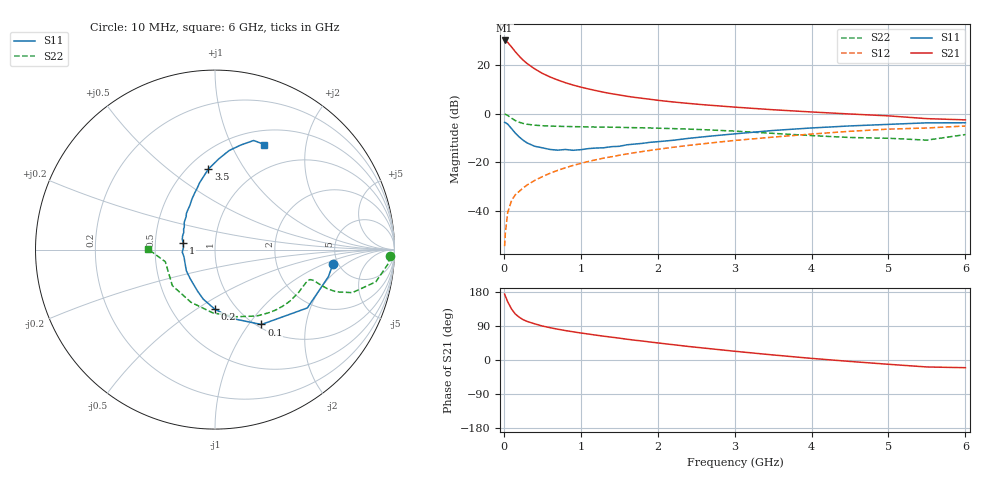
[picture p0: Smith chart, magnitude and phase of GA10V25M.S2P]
! Infineon Technologies  Discrete & RF Semiconductors
! BF775
! Si NPN RF Bipolar Junction Transistor in SOT23
! VCE = 10 V  IC = 25 mA
! Common Emitter S-Parameters:  May  1996
# GHz  S  MA  R  50
!  f  S11  S21  S12  S22
! GHz  MAG  ANG  MAG  ANG  MAG  ANG  MAG  ANG
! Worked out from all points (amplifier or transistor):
!   36 points, 10 MHz to 6 GHz, reference 50 ohm
!   highest |S21| = 30.0 dB at 10 MHz (marker M1)
!   |S21| within 3 dB of that: start of sweep to 108.8 MHz
!   unconditionally stable (mu >= 1): 401.8 MHz to 2.59 GHz
!   at 250 MHz: K = 0.86, MSG = 26.2 dB, |S12| = -30.5 dB
!   at 1.4 GHz: K = 1.10, MAG = 11.0 dB, |S12| = -17.7 dB
!   at 6 GHz: K = 0.90, MSG = 1.3 dB, |S12| = -5.1 dB
!   S11 on the Smith chart (normalised r, x): 10 MHz: 4.54, -1.29; 100 MHz: 1.05, -1.15; 200 MHz: 0.80, -0.59; 1 GHz: 0.70, +0.05; 3.5 GHz: 0.62, +0.70; 6 GHz: 0.67, +1.35
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0.01  0.6621 -6.9  31.6 173.9  0.0019 90.7  0.9771 -2.1
0.02  0.6498 -13.4  31.08 168.5  0.0036 81.0  0.9651 -5.0
0.05  0.6085 -32.3  28.86 153.7  0.0093 76.8  0.9143 -11.3
0.1  0.491 -58.2  23.3 134.5  0.0164 68.6  0.802 -17.4
0.15  0.3954 -76.0  18.48 121.2  0.0216 65.7  0.7162 -19.2
0.2  0.3307 -90.4  15.05 112.9  0.0253 66.3  0.6632 -19.2
0.25  0.2841 -103.2  12.49 106.5  0.0297 66.4  0.6271 -18.6
0.3  0.2509 -112.8  10.7 102.0  0.034 68.4  0.6042 -18.1
0.4  0.2132 -130.3  8.278 95.5  0.0423 70.0  0.5776 -17.4
0.5  0.1983 -143.7  6.683 89.7  0.0507 70.9  0.5619 -17.4
0.6  0.1833 -155.7  5.639 85.3  0.0594 71.1  0.5538 -17.6
0.7  0.1774 -167.2  4.884 81.3  0.0683 71.9  0.5476 -18.3
0.8  0.183 -175.4  4.293 77.7  0.0771 71.4  0.5432 -19.2
1  0.1812 168.2  3.487 71.3  0.0949 70.8  0.5358 -21.2
1.1  0.191 162.5  3.198 68.5  0.1041 70.4  0.532 -22.7
1.3  0.1985 151.4  2.732 62.8  0.1219 69.1  0.5266 -25.2
1.6  0.2285 138.6  2.263 54.8  0.1482 66.9  0.5162 -29.7
2.2  0.2827 119.8  1.729 40.4  0.2031 61.9  0.4907 -40.2
3.5  0.4493 94.8  1.197 13.3  0.3285 48.3  0.392 -72.6
4.5  0.5573 81.9  0.979 -3.8  0.4322 35.6  0.3225 -114.6
5.5  0.6449 70.5  0.786 -18.4  0.5055 19.5  0.2849 -166.3
6  0.6471 64.8  0.742 -20.3  0.5551 15.0  0.3707 179.8
